FUNCTION "FC_GRP_55" : VOID
TITLE =GROUP =55
{ S7_language := '9(1) Angielski (Stany Zjednoczone)  11.01.2022  09:45:15' }
VERSION : 0.1


VAR_TEMP
  CL : "UDT_CABINET";	//CABINET LOCAL
  CR : "UDT_CABINET";	//CABINET REMOTE
  RelError : BOOL ;	//ERROR RELEASE
  RelErrorCL : BOOL ;	//ERROR RELEASE FROM CABINET LOCAL
  RelErrorCR : BOOL ;	//ERROR RELEASE FROM CABINET REMOTE
  RelControl : BOOL ;	//CONTROL RELEASE
  RelControlCL : BOOL ;	//CONTROL RELEASE FROM CABINET LOCAL
  RelControlCR : BOOL ;	//CONTROL RELEASE FROM CABINET REMOTE
  ErrorConfirm : BOOL ;	//ERROR CONFIRM
  AutoOn : BOOL ;	//AUTOMATIC ON
  AutoOff : BOOL ;	//AUTOMATIC OFF
  RelAuto : BOOL ;	//AUTOMATIC RELEASE
  TempSetpoint : REAL ;
  dummy_bin : BOOL ;
END_VAR
BEGIN
NETWORK
TITLE =GLOBAL SIGNALS
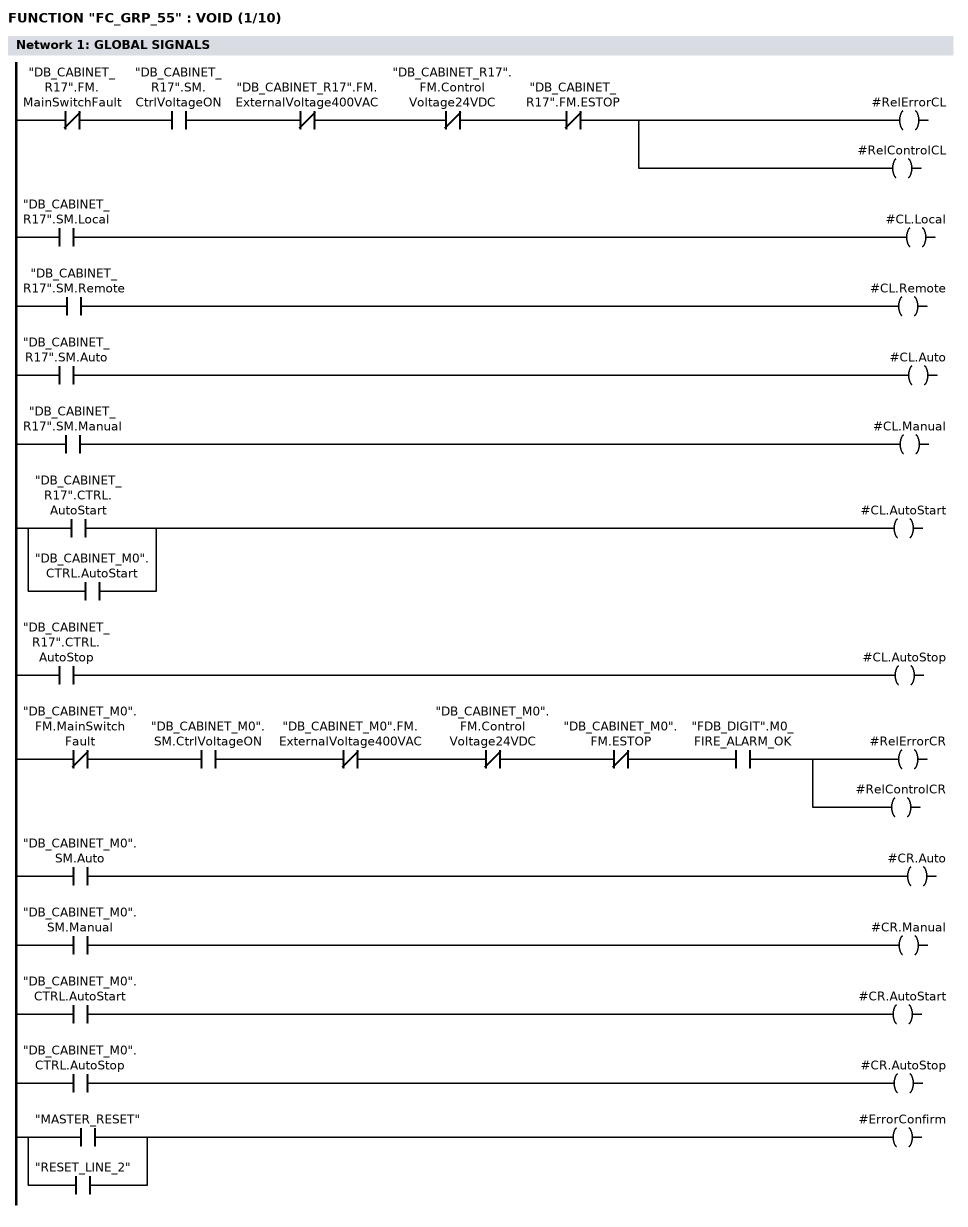
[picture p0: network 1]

//LOCAL
      UN    "DB_CABINET_R17".FM.MainSwitchFault;
      U     "DB_CABINET_R17".SM.CtrlVoltageON;
      UN    "DB_CABINET_R17".FM.ExternalVoltage400VAC;
      UN    "DB_CABINET_R17".FM.ControlVoltage24VDC;
      UN    "DB_CABINET_R17".FM.ESTOP;
      =     #RelErrorCL;
      =     #RelControlCL;

      U     "DB_CABINET_R17".SM.Local;
      =     #CL.Local;
      U     "DB_CABINET_R17".SM.Remote;
      =     #CL.Remote;
      U     "DB_CABINET_R17".SM.Auto;
      =     #CL.Auto;
      U     "DB_CABINET_R17".SM.Manual;
      =     #CL.Manual;
      U     "DB_CABINET_R17".CTRL.AutoStart;
      O     "DB_CABINET_M0".CTRL.AutoStart;
      =     #CL.AutoStart;
      U     "DB_CABINET_R17".CTRL.AutoStop;
      =     #CL.AutoStop;


//REMOTE

      UN    "DB_CABINET_M0".FM.MainSwitchFault;
      U     "DB_CABINET_M0".SM.CtrlVoltageON;
      UN    "DB_CABINET_M0".FM.ExternalVoltage400VAC;
      UN    "DB_CABINET_M0".FM.ControlVoltage24VDC;
//      UN    "DB_CABINET_M0".FM.ControlVoltage230VAC_MS
      UN    "DB_CABINET_M0".FM.ESTOP;
      U     "FDB_DIGIT".M0_FIRE_ALARM_OK;
      =     #RelErrorCR;
      =     #RelControlCR;

      U     "DB_CABINET_M0".SM.Auto;
      =     #CR.Auto;
      U     "DB_CABINET_M0".SM.Manual;
      =     #CR.Manual;
      U     "DB_CABINET_M0".CTRL.AutoStart;
      =     #CR.AutoStart;
      U     "DB_CABINET_M0".CTRL.AutoStop;
      =     #CR.AutoStop;


      U     "MASTER_RESET";
      O     "RESET_LINE_2";
      =     #ErrorConfirm;

NETWORK
TITLE =GLOBAL SIGNALS - GROUP GENERAL ERROR AND WARNING
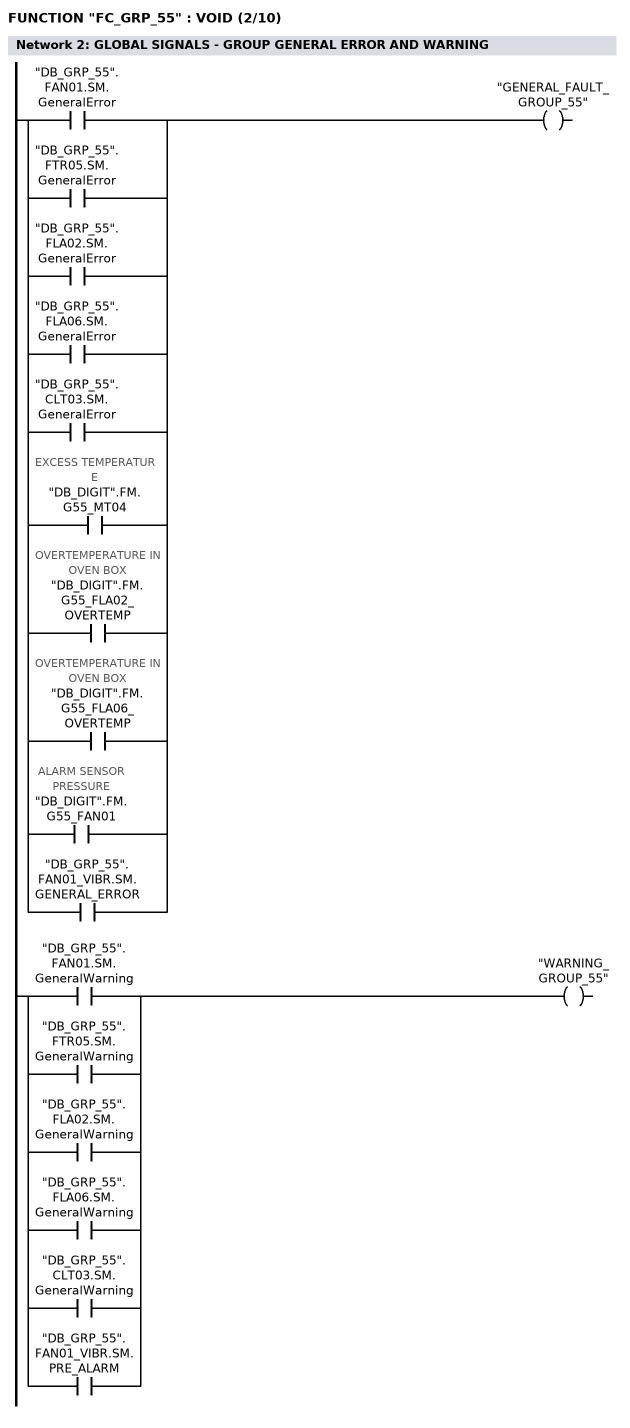
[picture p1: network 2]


      U     "DB_GRP_55".FAN01.SM.GeneralError;
      O     "DB_GRP_55".FTR05.SM.GeneralError;
      O     "DB_GRP_55".FLA02.SM.GeneralError;
      O     "DB_GRP_55".FLA06.SM.GeneralError;
      O     "DB_GRP_55".CLT03.SM.GeneralError;
      O     "DB_DIGIT".FM.G55_MT04; //EXCESS TEMPERATURE
      O     "DB_DIGIT".FM.G55_FLA02_OVERTEMP; //OVERTEMPERATURE IN OVEN BOX
      O     "DB_DIGIT".FM.G55_FLA06_OVERTEMP; //OVERTEMPERATURE IN OVEN BOX
      O     "DB_DIGIT".FM.G55_FAN01; //ALARM SENSOR PRESSURE
      O     "DB_GRP_55".FAN01_VIBR.SM.GENERAL_ERROR;
      =     "GENERAL_FAULT_GROUP_55";

      U     "DB_GRP_55".FAN01.SM.GeneralWarning;
      O     "DB_GRP_55".FTR05.SM.GeneralWarning;
      O     "DB_GRP_55".FLA02.SM.GeneralWarning;
      O     "DB_GRP_55".FLA06.SM.GeneralWarning;
      O     "DB_GRP_55".CLT03.SM.GeneralWarning;
      O     "DB_GRP_55".FAN01_VIBR.SM.PRE_ALARM;
      =     "WARNING_GROUP_55";


NETWORK
TITLE =RELEASE CONTROL
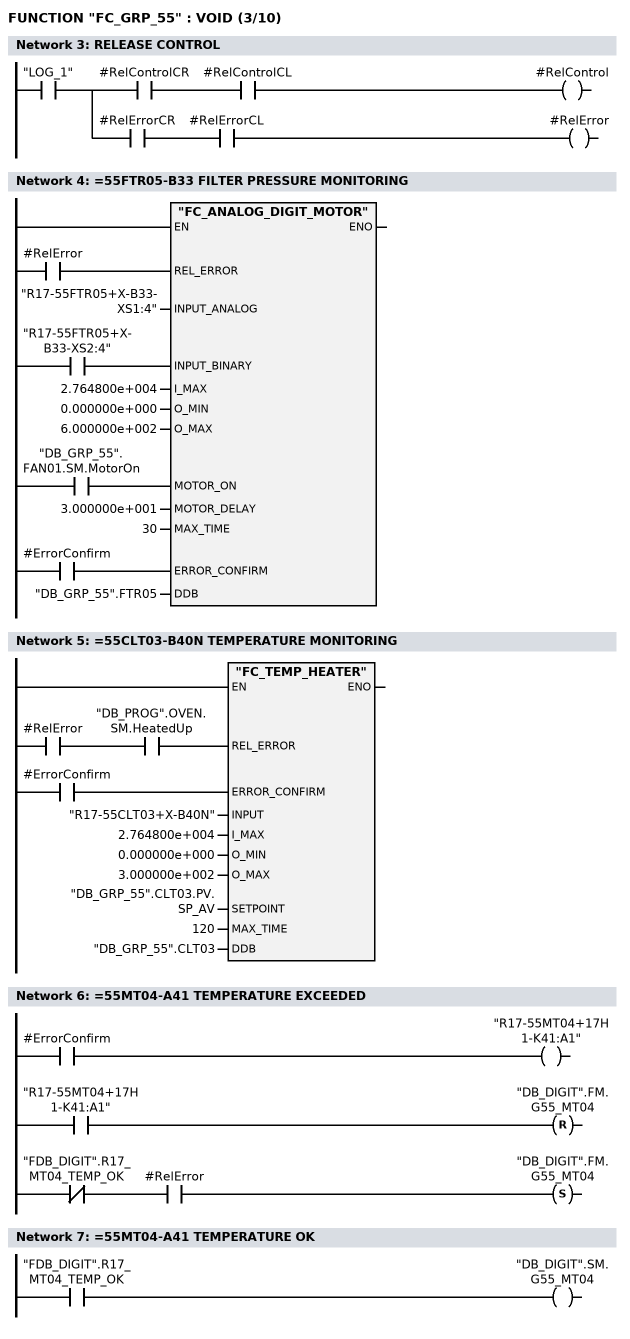
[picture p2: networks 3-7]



      U     "LOG_1";
      =     L     11.0;
      U     L     11.0;
      U     #RelControlCR;
      U     #RelControlCL;
      =     #RelControl;
      U     L     11.0;
      U     #RelErrorCR;
      U     #RelErrorCL;
      =     #RelError;
NETWORK
TITLE ==55FTR05-B33 FILTER PRESSURE MONITORING

      U     #RelError;
      =     L     11.0;
      BLD   103;
      U     "R17-55FTR05+X-B33-XS2:4";
      =     L     11.1;
      BLD   103;
      U     "DB_GRP_55".FAN01.SM.MotorOn;
      =     L     11.2;
      BLD   103;
      U     #ErrorConfirm;
      =     L     11.3;
      BLD   103;
      CALL "FC_ANALOG_DIGIT_MOTOR" (
           REL_ERROR                := L     11.0,
           INPUT_ANALOG             := "R17-55FTR05+X-B33-XS1:4",
           INPUT_BINARY             := L     11.1,
           I_MAX                    := 2.764800e+004,
           O_MIN                    := 0.000000e+000,
           O_MAX                    := 6.000000e+002,
           MOTOR_ON                 := L     11.2,
           MOTOR_DELAY              := 3.000000e+001,
           MAX_TIME                 := 30,
           ERROR_CONFIRM            := L     11.3,
           DDB                      := "DB_GRP_55".FTR05);
      NOP   0;
NETWORK
TITLE ==55CLT03-B40N TEMPERATURE MONITORING

      U     #RelError;
      U     "DB_PROG".OVEN.SM.HeatedUp;
      =     L     11.0;
      BLD   103;
      U     #ErrorConfirm;
      =     L     11.1;
      BLD   103;
      CALL "FC_TEMP_HEATER" (
           REL_ERROR                := L     11.0,
           ERROR_CONFIRM            := L     11.1,
           INPUT                    := "R17-55CLT03+X-B40N",
           I_MAX                    := 2.764800e+004,
           O_MIN                    := 0.000000e+000,
           O_MAX                    := 3.000000e+002,
           SETPOINT                 := "DB_GRP_55".CLT03.PV.SP_AV,
           MAX_TIME                 := 120,
           DDB                      := "DB_GRP_55".CLT03);
      NOP   0;
NETWORK
TITLE ==55MT04-A41 TEMPERATURE EXCEEDED

      U     #ErrorConfirm;
      =     "R17-55MT04+17H1-K41:A1";
      U     "R17-55MT04+17H1-K41:A1";
      R     "DB_DIGIT".FM.G55_MT04;
      UN    "FDB_DIGIT".R17_MT04_TEMP_OK;
      U     #RelError;
      S     "DB_DIGIT".FM.G55_MT04;
      NOP   0;
NETWORK
TITLE ==55MT04-A41 TEMPERATURE OK

      U     "FDB_DIGIT".R17_MT04_TEMP_OK;
      =     "DB_DIGIT".SM.G55_MT04;
NETWORK
TITLE ==55MT04-A41 OVERTEMPERATURE FAULT RESET
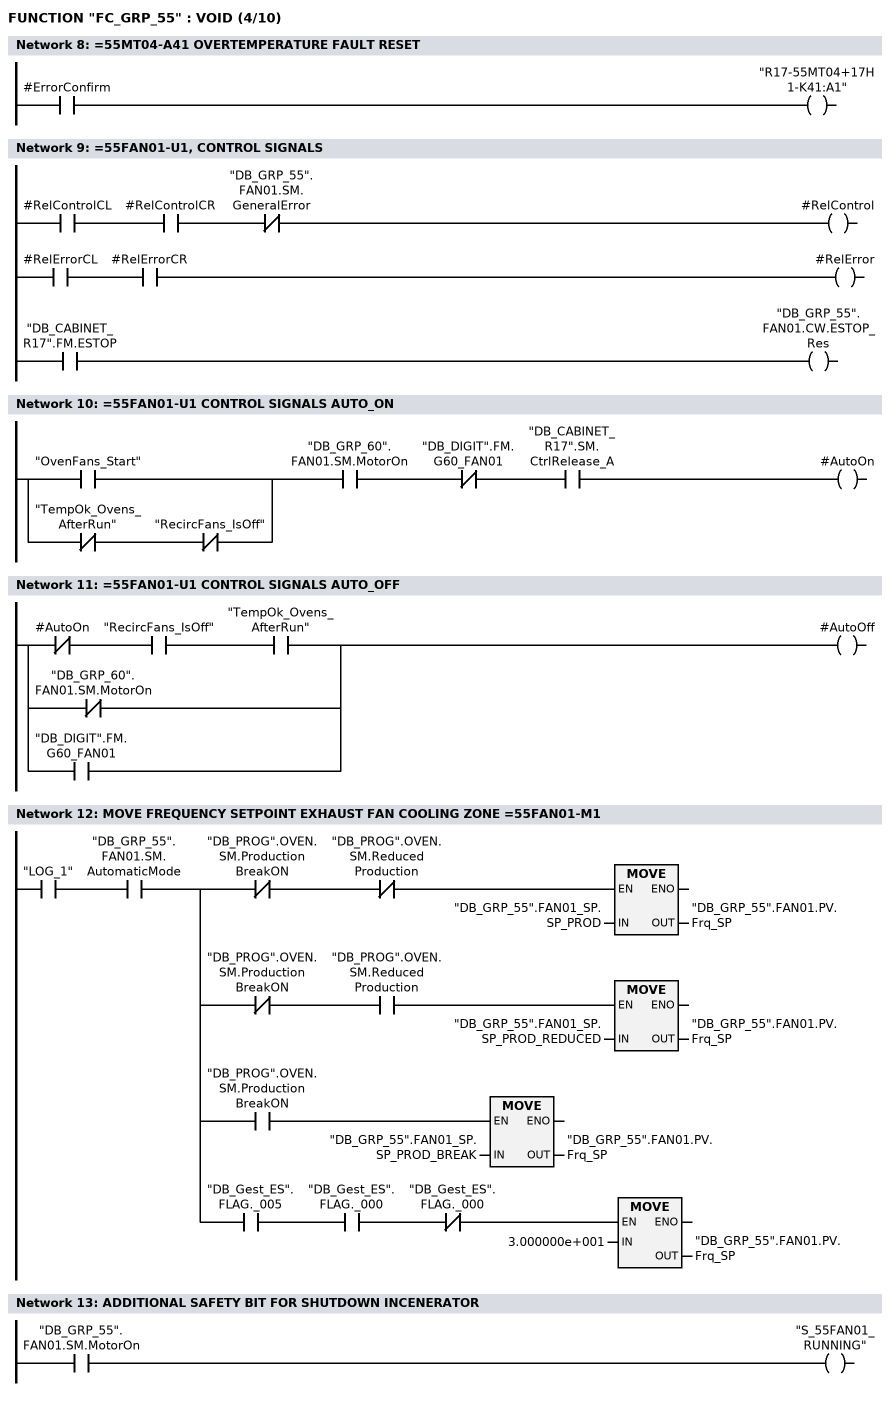
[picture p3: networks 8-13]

      U     #ErrorConfirm;
      =     "R17-55MT04+17H1-K41:A1";
NETWORK
TITLE ==55FAN01-U1, CONTROL SIGNALS

      U     #RelControlCL;
      U     #RelControlCR;
      UN    "DB_GRP_55".FAN01.SM.GeneralError;
      =     #RelControl;


      U     #RelErrorCL;
      U     #RelErrorCR;
      =     #RelError;

      U     "DB_CABINET_R17".FM.ESTOP;
      =     "DB_GRP_55".FAN01.CW.ESTOP_Res;

NETWORK
TITLE ==55FAN01-U1 CONTROL SIGNALS AUTO_ON

      U(    ;
      O     "OvenFans_Start";
      O     ;
      UN    "TempOk_Ovens_AfterRun";
      UN    "RecircFans_IsOff";
      )     ;
      U     "DB_GRP_60".FAN01.SM.MotorOn;
      UN    "DB_DIGIT".FM.G60_FAN01;
      U     "DB_CABINET_R17".SM.CtrlRelease_A;
      =     #AutoOn;
NETWORK
TITLE ==55FAN01-U1 CONTROL SIGNALS AUTO_OFF

      UN    #AutoOn;
      U     "RecircFans_IsOff";
      U     "TempOk_Ovens_AfterRun";
      ON    "DB_GRP_60".FAN01.SM.MotorOn;
      O     "DB_DIGIT".FM.G60_FAN01;
      =     #AutoOff;
NETWORK
TITLE =MOVE FREQUENCY SETPOINT EXHAUST FAN COOLING ZONE =55FAN01-M1

      U     "LOG_1";
      U     "DB_GRP_55".FAN01.SM.AutomaticMode;
      =     L     11.0;
      U     L     11.0;
      UN    "DB_PROG".OVEN.SM.ProductionBreakON;
      UN    "DB_PROG".OVEN.SM.ReducedProduction;
      SPBNB _001;
      L     "DB_GRP_55".FAN01_SP.SP_PROD;
      T     "DB_GRP_55".FAN01.PV.Frq_SP;
_001: NOP   0;
      U     L     11.0;
      UN    "DB_PROG".OVEN.SM.ProductionBreakON;
      U     "DB_PROG".OVEN.SM.ReducedProduction;
      SPBNB _002;
      L     "DB_GRP_55".FAN01_SP.SP_PROD_REDUCED;
      T     "DB_GRP_55".FAN01.PV.Frq_SP;
_002: NOP   0;
      U     L     11.0;
      U     "DB_PROG".OVEN.SM.ProductionBreakON;
      SPBNB _003;
      L     "DB_GRP_55".FAN01_SP.SP_PROD_BREAK;
      T     "DB_GRP_55".FAN01.PV.Frq_SP;
_003: NOP   0;
      U     L     11.0;
      U     "DB_Gest_ES".FLAG._005;
      U     "DB_Gest_ES".FLAG._000;
      UN    "DB_Gest_ES".FLAG._000;
      SPBNB _004;
      L     3.000000e+001;
      T     "DB_GRP_55".FAN01.PV.Frq_SP;
_004: NOP   0;
NETWORK
TITLE =ADDITIONAL SAFETY BIT FOR SHUTDOWN INCENERATOR

      U     "DB_GRP_55".FAN01.SM.MotorOn;
      =     "S_55FAN01_RUNNING";
NETWORK
TITLE =COAST DOWN ENABLED 55FAN01
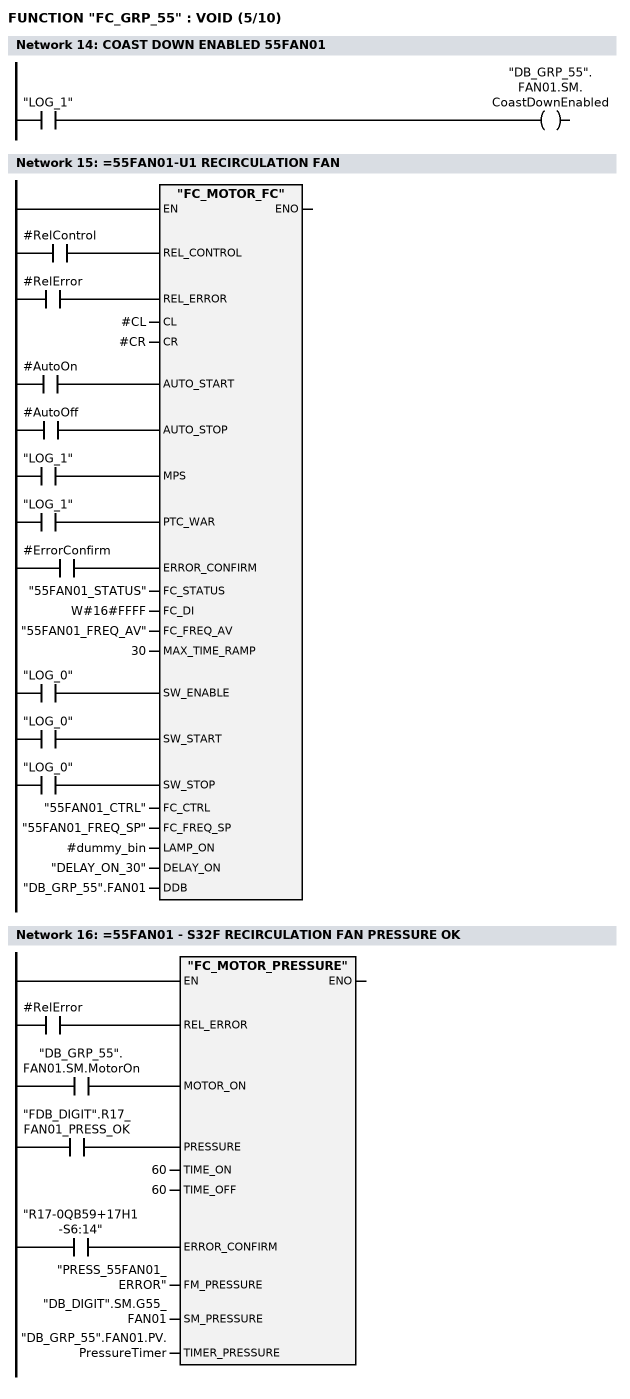
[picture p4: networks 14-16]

      U     "LOG_1";
      =     "DB_GRP_55".FAN01.SM.CoastDownEnabled;
NETWORK
TITLE ==55FAN01-U1 RECIRCULATION FAN

      U     #RelControl;
      =     L     11.0;
      BLD   103;
      U     #RelError;
      =     L     11.1;
      BLD   103;
      U     #AutoOn;
      =     L     11.2;
      BLD   103;
      U     #AutoOff;
      =     L     11.3;
      BLD   103;
      U     "LOG_1";
      =     L     11.4;
      BLD   103;
      U     "LOG_1";
      =     L     11.5;
      BLD   103;
      U     #ErrorConfirm;
      =     L     11.6;
      BLD   103;
      U     "LOG_0";
      =     L     11.7;
      BLD   103;
      U     "LOG_0";
      =     L     12.0;
      BLD   103;
      U     "LOG_0";
      =     L     12.1;
      BLD   103;
      CALL "FC_MOTOR_FC" (
           REL_CONTROL              := L     11.0,
           REL_ERROR                := L     11.1,
           CL                       := #CL,
           CR                       := #CR,
           AUTO_START               := L     11.2,
           AUTO_STOP                := L     11.3,
           MPS                      := L     11.4,
           PTC_WAR                  := L     11.5,
           ERROR_CONFIRM            := L     11.6,
           FC_STATUS                := "55FAN01_STATUS",
           FC_DI                    := W#16#FFFF,
           FC_FREQ_AV               := "55FAN01_FREQ_AV",
           MAX_TIME_RAMP            := 30,
           SW_ENABLE                := L     11.7,
           SW_START                 := L     12.0,
           SW_STOP                  := L     12.1,
           FC_CTRL                  := "55FAN01_CTRL",
           FC_FREQ_SP               := "55FAN01_FREQ_SP",
           LAMP_ON                  := #dummy_bin,
           DELAY_ON                 := "DELAY_ON_30",
           DDB                      := "DB_GRP_55".FAN01);
      NOP   0;
NETWORK
TITLE ==55FAN01 - S32F RECIRCULATION FAN PRESSURE OK

      U     #RelError;
      =     L     11.0;
      BLD   103;
      U     "DB_GRP_55".FAN01.SM.MotorOn;
      =     L     11.1;
      BLD   103;
      U     "FDB_DIGIT".R17_FAN01_PRESS_OK;
      =     L     11.2;
      BLD   103;
      U     "R17-0QB59+17H1-S6:14";
      =     L     11.3;
      BLD   103;
      CALL "FC_MOTOR_PRESSURE" (
           REL_ERROR                := L     11.0,
           MOTOR_ON                 := L     11.1,
           PRESSURE                 := L     11.2,
           TIME_ON                  := 60,
           TIME_OFF                 := 60,
           ERROR_CONFIRM            := L     11.3,
           FM_PRESSURE              := "PRESS_55FAN01_ERROR",
           SM_PRESSURE              := "DB_DIGIT".SM.G55_FAN01,
           TIMER_PRESSURE           := "DB_GRP_55".FAN01.PV.PressureTimer);
      NOP   0;
NETWORK
TITLE =PRESSURE ERROR =55FAN01
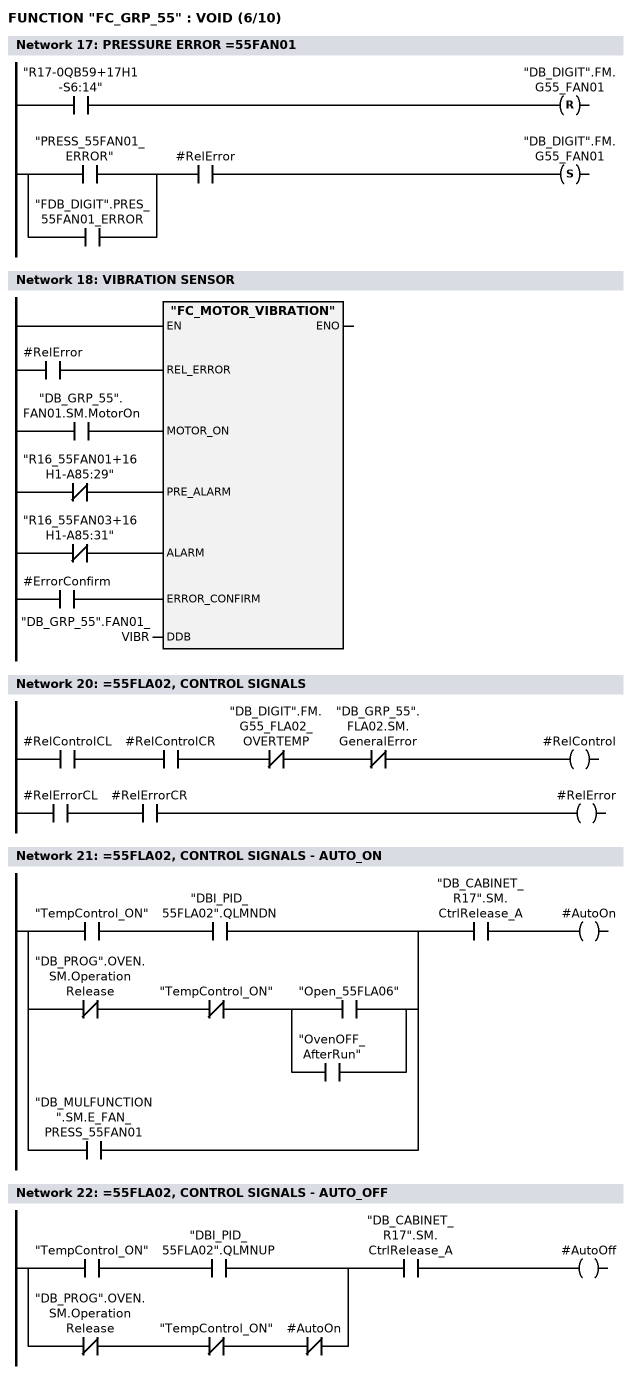
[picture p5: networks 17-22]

      U     "R17-0QB59+17H1-S6:14";
      R     "DB_DIGIT".FM.G55_FAN01;
      U(    ;
      O     "PRESS_55FAN01_ERROR";
      O     "FDB_DIGIT".PRES_55FAN01_ERROR;
      )     ;
      U     #RelError;
      S     "DB_DIGIT".FM.G55_FAN01;
      NOP   0;
NETWORK
TITLE =VIBRATION SENSOR

      U     #RelError;
      =     L     11.0;
      BLD   103;
      U     "DB_GRP_55".FAN01.SM.MotorOn;
      =     L     11.1;
      BLD   103;
      UN    "R16_55FAN01+16H1-A85:29";
      =     L     11.2;
      BLD   103;
      UN    "R16_55FAN03+16H1-A85:31";
      =     L     11.3;
      BLD   103;
      U     #ErrorConfirm;
      =     L     11.4;
      BLD   103;
      CALL "FC_MOTOR_VIBRATION" (
           REL_ERROR                := L     11.0,
           MOTOR_ON                 := L     11.1,
           PRE_ALARM                := L     11.2,
           ALARM                    := L     11.3,
           ERROR_CONFIRM            := L     11.4,
           DDB                      := "DB_GRP_55".FAN01_VIBR);
      NOP   0;
NETWORK
TITLE =********* 55FLA02 ***********

NETWORK
TITLE ==55FLA02, CONTROL SIGNALS

      U     #RelControlCL;
      U     #RelControlCR;
      UN    "DB_DIGIT".FM.G55_FLA02_OVERTEMP;
      UN    "DB_GRP_55".FLA02.SM.GeneralError;
      =     #RelControl;



      U     #RelErrorCL;
      U     #RelErrorCR;
      =     #RelError;


NETWORK
TITLE ==55FLA02, CONTROL SIGNALS - AUTO_ON

      U(    ;
      U     "TempControl_ON";
      U     "DBI_PID_55FLA02".QLMNDN;
      O     ;
      UN    "DB_PROG".OVEN.SM.OperationRelease;
      UN    "TempControl_ON";
      U(    ;
      O     "Open_55FLA06";
      O     "OvenOFF_AfterRun";
      )     ;
      O     "DB_MULFUNCTION".SM.E_FAN_PRESS_55FAN01;
      )     ;
      U     "DB_CABINET_R17".SM.CtrlRelease_A;
      =     #AutoOn;
NETWORK
TITLE ==55FLA02, CONTROL SIGNALS - AUTO_OFF

      U(    ;
      U     "TempControl_ON";
      U     "DBI_PID_55FLA02".QLMNUP;
      O     ;
      UN    "DB_PROG".OVEN.SM.OperationRelease;
      UN    "TempControl_ON";
      UN    #AutoOn;
      )     ;
      U     "DB_CABINET_R17".SM.CtrlRelease_A;
      =     #AutoOff;
NETWORK
TITLE =FIRE ALARM OPEN
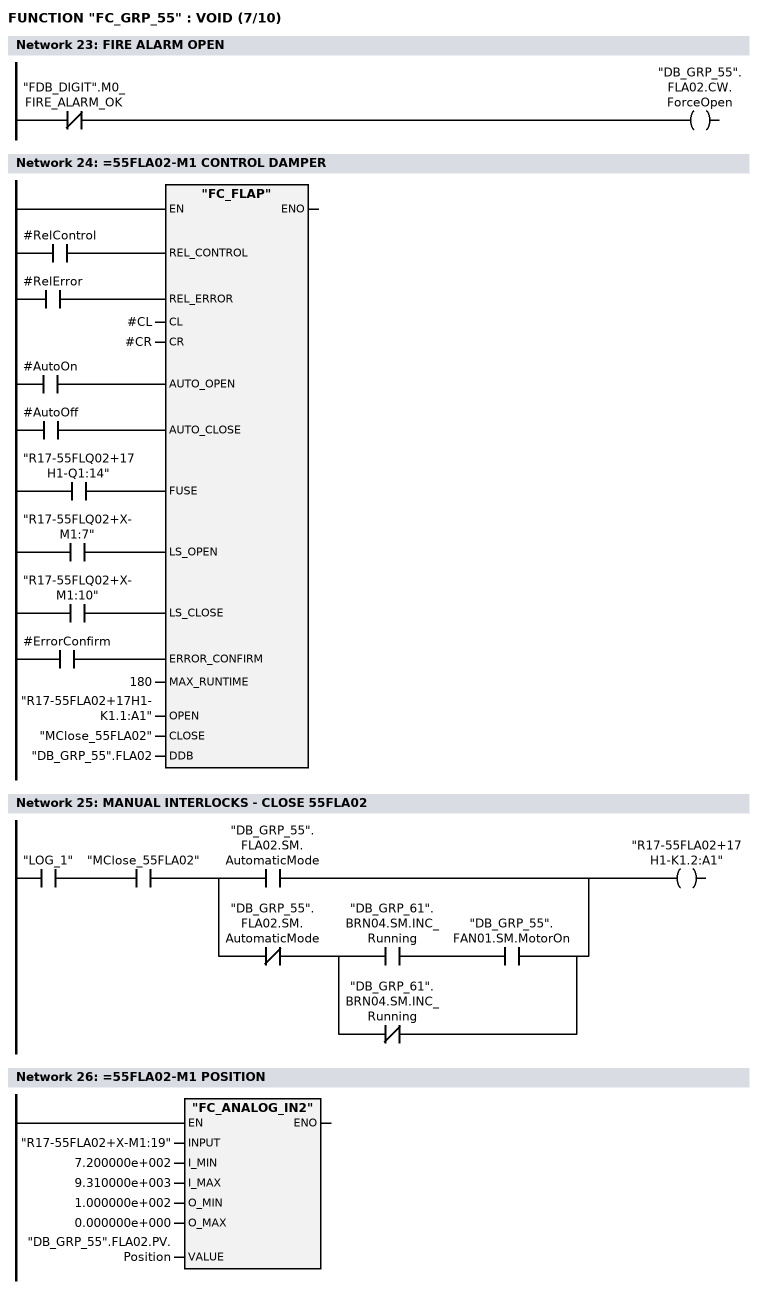
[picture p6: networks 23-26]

      UN    "FDB_DIGIT".M0_FIRE_ALARM_OK;
      =     "DB_GRP_55".FLA02.CW.ForceOpen;
NETWORK
TITLE ==55FLA02-M1 CONTROL DAMPER



      U     #RelControl;
      =     L     11.0;
      BLD   103;
      U     #RelError;
      =     L     11.1;
      BLD   103;
      U     #AutoOn;
      =     L     11.2;
      BLD   103;
      U     #AutoOff;
      =     L     11.3;
      BLD   103;
      U     "R17-55FLQ02+17H1-Q1:14";
      =     L     11.4;
      BLD   103;
      U     "R17-55FLQ02+X-M1:7";
      =     L     11.5;
      BLD   103;
      U     "R17-55FLQ02+X-M1:10";
      =     L     11.6;
      BLD   103;
      U     #ErrorConfirm;
      =     L     11.7;
      BLD   103;
      CALL "FC_FLAP" (
           REL_CONTROL              := L     11.0,
           REL_ERROR                := L     11.1,
           CL                       := #CL,
           CR                       := #CR,
           AUTO_OPEN                := L     11.2,
           AUTO_CLOSE               := L     11.3,
           FUSE                     := L     11.4,
           LS_OPEN                  := L     11.5,
           LS_CLOSE                 := L     11.6,
           ERROR_CONFIRM            := L     11.7,
           MAX_RUNTIME              := 180,
           OPEN                     := "R17-55FLA02+17H1-K1.1:A1",
           CLOSE                    := "MClose_55FLA02",
           DDB                      := "DB_GRP_55".FLA02);
      NOP   0;
NETWORK
TITLE =MANUAL INTERLOCKS - CLOSE 55FLA02

      U     "LOG_1";
      U     "MClose_55FLA02";
      U(    ;
      O     "DB_GRP_55".FLA02.SM.AutomaticMode;
      O     ;
      UN    "DB_GRP_55".FLA02.SM.AutomaticMode;
      U(    ;
      U     "DB_GRP_61".BRN04.SM.INC_Running;
      U     "DB_GRP_55".FAN01.SM.MotorOn;
      ON    "DB_GRP_61".BRN04.SM.INC_Running;
      )     ;
      )     ;
      =     "R17-55FLA02+17H1-K1.2:A1";
NETWORK
TITLE ==55FLA02-M1 POSITION

      CALL "FC_ANALOG_IN2" (
           INPUT                    := "R17-55FLA02+X-M1:19",
           I_MIN                    := 7.200000e+002,
           I_MAX                    := 9.310000e+003,
           O_MIN                    := 1.000000e+002,
           O_MAX                    := 0.000000e+000,
           VALUE                    := "DB_GRP_55".FLA02.PV.Position);
      NOP   0;
NETWORK
TITLE ==55FLA02-M1 TEMPERATURE FAULT
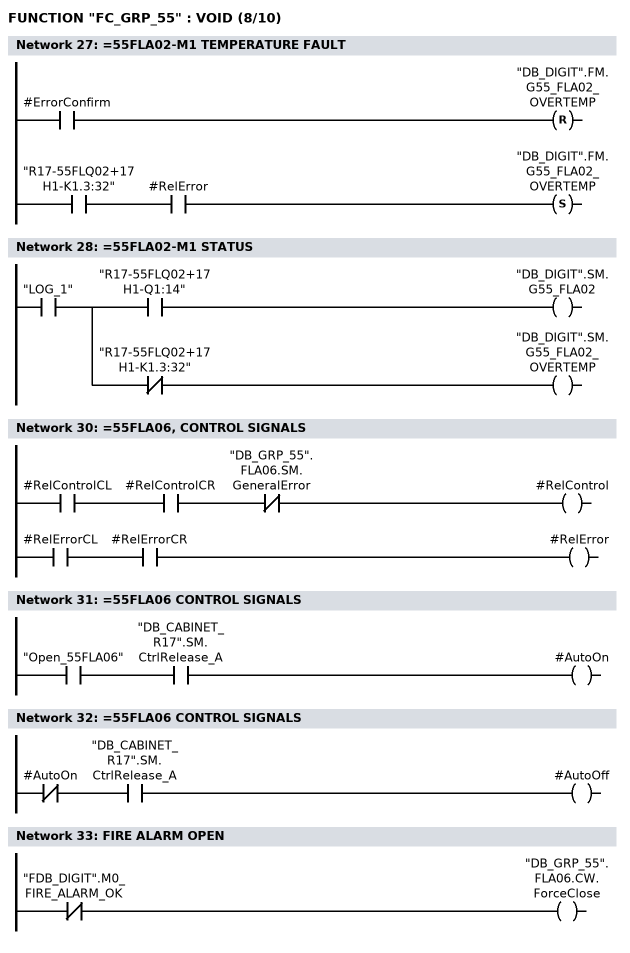
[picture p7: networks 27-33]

      U     #ErrorConfirm;
      R     "DB_DIGIT".FM.G55_FLA02_OVERTEMP;
      U     "R17-55FLQ02+17H1-K1.3:32";
      U     #RelError;
      S     "DB_DIGIT".FM.G55_FLA02_OVERTEMP;
      NOP   0;
NETWORK
TITLE ==55FLA02-M1 STATUS

      U     "LOG_1";
      =     L     11.0;
      U     L     11.0;
      U     "R17-55FLQ02+17H1-Q1:14";
      =     "DB_DIGIT".SM.G55_FLA02;
      U     L     11.0;
      UN    "R17-55FLQ02+17H1-K1.3:32";
      =     "DB_DIGIT".SM.G55_FLA02_OVERTEMP;
NETWORK
TITLE =********** 55LFA06 **************

NETWORK
TITLE ==55FLA06, CONTROL SIGNALS

      U     #RelControlCL;
      U     #RelControlCR;
      UN    "DB_GRP_55".FLA06.SM.GeneralError;
      =     #RelControl;


      U     #RelErrorCL;
      U     #RelErrorCR;
      =     #RelError;





NETWORK
TITLE ==55FLA06 CONTROL SIGNALS

      U     "Open_55FLA06";
      U     "DB_CABINET_R17".SM.CtrlRelease_A;
      =     #AutoOn;
NETWORK
TITLE ==55FLA06 CONTROL SIGNALS

      UN    #AutoOn;
      U     "DB_CABINET_R17".SM.CtrlRelease_A;
      =     #AutoOff;
NETWORK
TITLE =FIRE ALARM OPEN

      UN    "FDB_DIGIT".M0_FIRE_ALARM_OK;
      =     "DB_GRP_55".FLA06.CW.ForceClose;
NETWORK
TITLE ==55FLA06-M1 CONTROL DAMPER
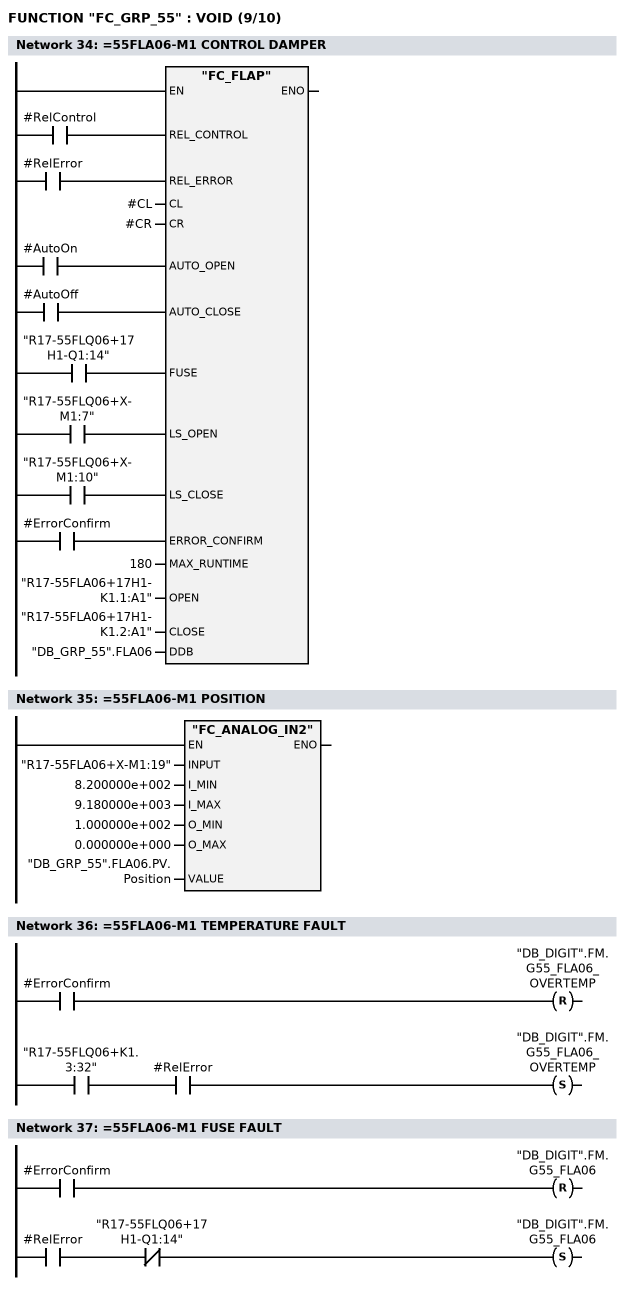
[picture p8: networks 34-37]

      U     #RelControl;
      =     L     11.0;
      BLD   103;
      U     #RelError;
      =     L     11.1;
      BLD   103;
      U     #AutoOn;
      =     L     11.2;
      BLD   103;
      U     #AutoOff;
      =     L     11.3;
      BLD   103;
      U     "R17-55FLQ06+17H1-Q1:14";
      =     L     11.4;
      BLD   103;
      U     "R17-55FLQ06+X-M1:7";
      =     L     11.5;
      BLD   103;
      U     "R17-55FLQ06+X-M1:10";
      =     L     11.6;
      BLD   103;
      U     #ErrorConfirm;
      =     L     11.7;
      BLD   103;
      CALL "FC_FLAP" (
           REL_CONTROL              := L     11.0,
           REL_ERROR                := L     11.1,
           CL                       := #CL,
           CR                       := #CR,
           AUTO_OPEN                := L     11.2,
           AUTO_CLOSE               := L     11.3,
           FUSE                     := L     11.4,
           LS_OPEN                  := L     11.5,
           LS_CLOSE                 := L     11.6,
           ERROR_CONFIRM            := L     11.7,
           MAX_RUNTIME              := 180,
           OPEN                     := "R17-55FLA06+17H1-K1.1:A1",
           CLOSE                    := "R17-55FLA06+17H1-K1.2:A1",
           DDB                      := "DB_GRP_55".FLA06);
      NOP   0;
NETWORK
TITLE ==55FLA06-M1 POSITION

      CALL "FC_ANALOG_IN2" (
           INPUT                    := "R17-55FLA06+X-M1:19",
           I_MIN                    := 8.200000e+002,
           I_MAX                    := 9.180000e+003,
           O_MIN                    := 1.000000e+002,
           O_MAX                    := 0.000000e+000,
           VALUE                    := "DB_GRP_55".FLA06.PV.Position);
      NOP   0;
NETWORK
TITLE ==55FLA06-M1 TEMPERATURE FAULT

      U     #ErrorConfirm;
      R     "DB_DIGIT".FM.G55_FLA06_OVERTEMP;
      U     "R17-55FLQ06+K1.3:32";
      U     #RelError;
      S     "DB_DIGIT".FM.G55_FLA06_OVERTEMP;
      NOP   0;
NETWORK
TITLE ==55FLA06-M1 FUSE FAULT

      U     #ErrorConfirm;
      R     "DB_DIGIT".FM.G55_FLA06;
      U     #RelError;
      UN    "R17-55FLQ06+17H1-Q1:14";
      S     "DB_DIGIT".FM.G55_FLA06;
      NOP   0;
NETWORK
TITLE ==55FLA06-M1 STATUS
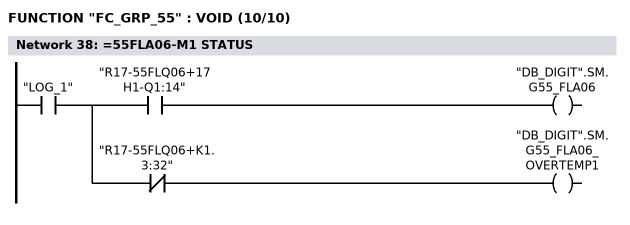
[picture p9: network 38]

      U     "LOG_1";
      =     L     11.0;
      U     L     11.0;
      U     "R17-55FLQ06+17H1-Q1:14";
      =     "DB_DIGIT".SM.G55_FLA06;
      U     L     11.0;
      UN    "R17-55FLQ06+K1.3:32";
      =     "DB_DIGIT".SM.G55_FLA06_OVERTEMP1;
NETWORK
TITLE =END

END_FUNCTION

